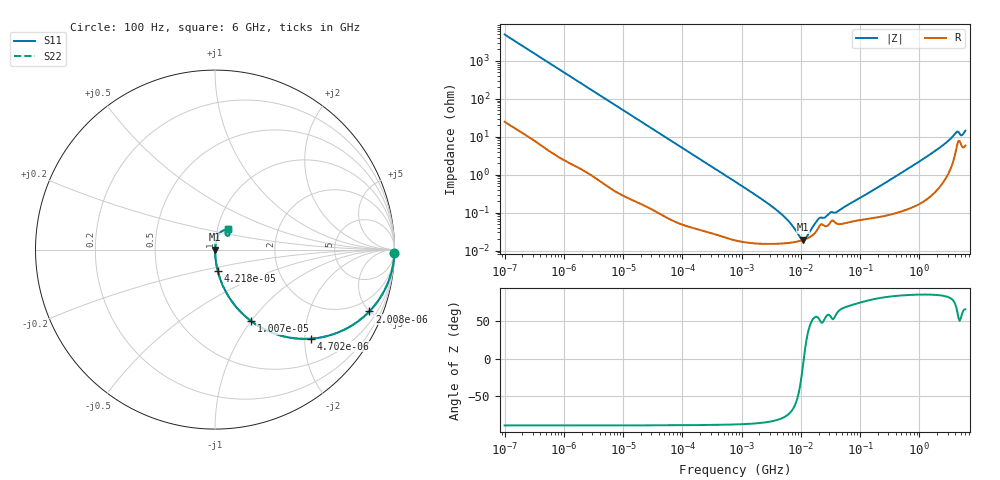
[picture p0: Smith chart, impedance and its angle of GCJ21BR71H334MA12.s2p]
!Murata Part Number: GCJ21BR71H334MA12
!These Parameters are Measured in Series Mode Connection
!Data Generated on Mar 13, 2026
!  o--ll--o
!Port1  Port2
!  o------o
!Operation Temp=25[degC], DC Bias Voltage=0[V]
!Freq. Start=100[Hz] Stop=6[GHz] 401[Steps]
# Hz S RI R 50
!Freq.(Hz) S11(Real) S11(Imag) S21(Real) S21(Imag) S12(Real) S12(Imag) S22(Real) S22(Imag)
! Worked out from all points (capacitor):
!   401 points, 100 Hz to 6 GHz, reference 50 ohm
!   read as one part in series: C = 321 nF near 109 Hz
!   lowest |Z| = 19.3 mohm at 10.87 MHz (marker M1)
!   series resonance near 11.24 MHz, so ESL is about 630 pH
!   S11 on the Smith chart (normalised r, x): 100 Hz: open; 2.008 kHz: 1.03, -4.98; 4.702 kHz: 1.01, -2.14; 10.07 kHz: 1.01, -1.00; 42.18 kHz: 1.00, -0.24; 6 GHz: 1.12, +0.26
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100  0.9995 -0.0202  0.000508 0.0202  0.000508 0.0202  0.9995 -0.0202
548  0.9875 -0.1085  0.0125 0.1085  0.0125 0.1085  0.9875 -0.1085
2008  0.8599 -0.3444  0.1401 0.3444  0.1401 0.3444  0.8599 -0.3444
4702  0.5325 -0.4963  0.4675 0.4963  0.4675 0.4963  0.5325 -0.4963
10066  0.2012 -0.3981  0.7988 0.3981  0.7988 0.3981  0.2012 -0.3981
18016  0.074 -0.2586  0.926 0.2586  0.926 0.2586  0.074 -0.2586
40335  0.0164 -0.1232  0.9836 0.1232  0.9836 0.1232  0.0164 -0.1232
42182  0.0151 -0.118  0.9849 0.118  0.9849 0.118  0.0151 -0.118
774597  0.00023 -0.0066  0.9998 0.0066  0.9998 0.0066  0.00023 -0.0066
4246196  0.000153 -0.00104  0.9998 0.00104  0.9998 0.00104  0.000153 -0.00104
6353432  0.00016 -0.000552  0.9998 0.000552  0.9998 0.000552  0.00016 -0.000552
9506416  0.000179 -0.000155  0.9998 0.000155  0.9998 0.000155  0.000179 -0.000155
1.087309e7  0.00019 -3.06e-05  0.9998 3.06e-05  0.9998 3.06e-05  0.00019 -3.06e-05
1.243624e7  0.000206 9.38e-05  0.9998 -9.38e-05  0.9998 -9.38e-05  0.000206 9.38e-05
1.555665e7  0.00025 0.000311  0.9997 -0.000311  0.9997 -0.000311  0.00025 0.000311
2.035112e7  0.000428 0.000568  0.9996 -0.000568  0.9996 -0.000568  0.000428 0.000568
4.165952e7  0.000504 0.000947  0.9995 -0.000947  0.9995 -0.000947  0.000504 0.000947
3.124326e8  0.000923 0.00705  0.9991 -0.00705  0.9991 -0.00705  0.000923 0.00705
1.873145e9  0.00533 0.0424  0.9947 -0.0424  0.9947 -0.0424  0.00533 0.0424
4.193612e9  0.0568 0.1094  0.9432 -0.1094  0.9432 -0.1094  0.0568 0.1094
5.245841e9  0.0601 0.0841  0.9399 -0.0841  0.9399 -0.0841  0.0601 0.0841
6e9  0.0701 0.1157  0.9299 -0.1157  0.9299 -0.1157  0.0701 0.1157
